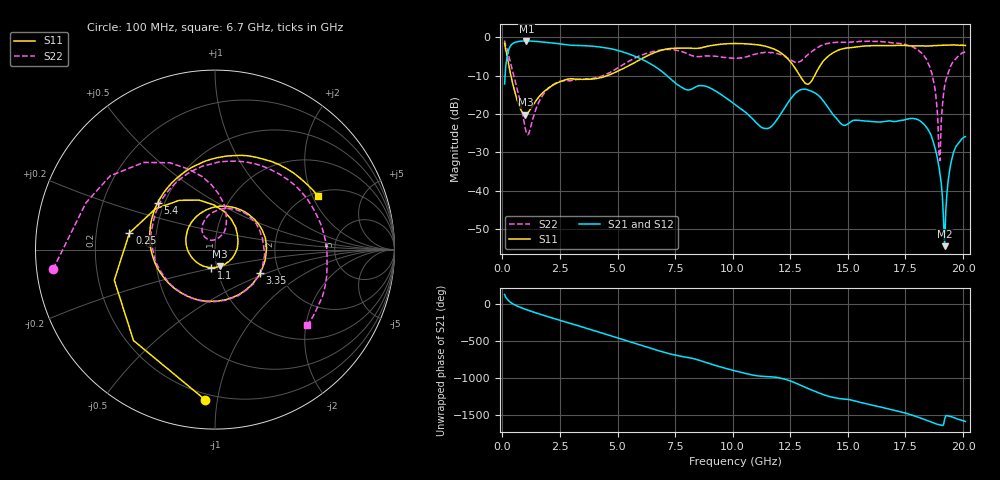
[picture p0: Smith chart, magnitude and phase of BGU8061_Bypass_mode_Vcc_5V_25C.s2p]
# GHZ S DB R 50
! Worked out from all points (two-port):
!   401 points, 100 MHz to 20.1 GHz, reference 50 ohm
!   highest |S21| = -0.96 dB at 1.05 GHz (marker M1); lowest = -54.5 dB at 19.2 GHz (marker M2)
!   |S21| within 3 dB of the highest: 245.2 MHz to 5.305 GHz (5.06 GHz wide, 182 % of centre)
!   lowest |S11| = -20.2 dB at 1 GHz (marker M3), VSWR 1.22, Z = 52 - j9.77 ohm
!   |S11| at or under -10 dB: 372.1 MHz to 4.568 GHz (4.196 GHz wide, 170 % of centre); 12.91 GHz to 13.56 GHz (642.8 MHz wide, 4.86 % of centre)
!   |S22| runs from -32.2 to -0.8 dB; largest |S21 - S12| = 0.014
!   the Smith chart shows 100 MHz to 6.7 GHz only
!   S11 on the Smith chart (normalised r, x): 100 MHz: 0.16, -0.93; 250 MHz: 0.35, +0.08; 1.1 GHz: 0.94, -0.19; 3.35 GHz: 1.60, -0.44; 5.4 GHz: 0.46, +0.29; 6.7 GHz: 2.16, +2.20
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0.1  -1.51 -93.6  -12.18 126.3  -12.16 126.3  -0.84 -173.2
0.25  -6.27 169.0  -3.80 51.1  -3.80 51.1  -4.05 129.3
1  -20.23 -72.7  -0.97 -72.8  -1.01 -73.2  -23.84 75.2
1.05  -20.08 -87.9  -0.96 -78.3  -1.00 -78.7  -25.00 85.9
1.1  -19.77 -101.2  -0.97 -83.9  -1.01 -84.2  -25.43 99.0
2.1  -12.85 100.8  -1.46 175.8  -1.49 175.5  -12.78 80.4
3.35  -10.98 -26.9  -2.15 59.7  -2.17 59.2  -10.93 -30.9
3.45  -10.98 -36.1  -2.17 50.3  -2.20 49.8  -10.84 -41.2
5.4  -7.71 141.1  -4.15 -139.8  -4.19 -139.6  -6.55 98.4
6.7  -3.80 27.3  -7.94 95.0  -7.96 94.6  -3.53 -39.3
6.8  -3.60 18.5  -8.35 85.7  -8.37 85.3  -3.39 -49.5
8  -2.83 -75.0  -13.69 -1.5  -13.70 -1.8  -4.21 -171.7
9.1  -2.14 -141.1  -13.47 -97.8  -13.50 -97.4  -4.88 89.0
10.1  -1.63 158.9  -17.56 174.8  -17.60 174.9  -5.44 -29.4
12.15  -4.30 32.1  -19.41 71.6  -19.40 71.8  -4.69 135.6
13.45  -11.15 -155.3  -14.18 -87.5  -14.19 -87.7  -3.62 102.7
14.7  -3.12 72.6  -22.54 157.9  -22.57 157.6  -1.33 42.2
16.8  -2.18 -25.1  -21.78 16.9  -21.84 19.0  -1.33 -46.7
18.5  -2.27 -90.7  -24.26 -143.7  -24.20 -143.4  -7.01 -154.3
18.95  -2.13 -108.5  -33.70 166.3  -33.70 167.0  -30.07 131.3
19.2  -2.07 -118.7  -54.49 -117.1  -54.78 -122.8  -12.66 -45.2
20.1  -2.14 -157.3  -25.92 -148.4  -25.95 -148.3  -3.76 -122.2
